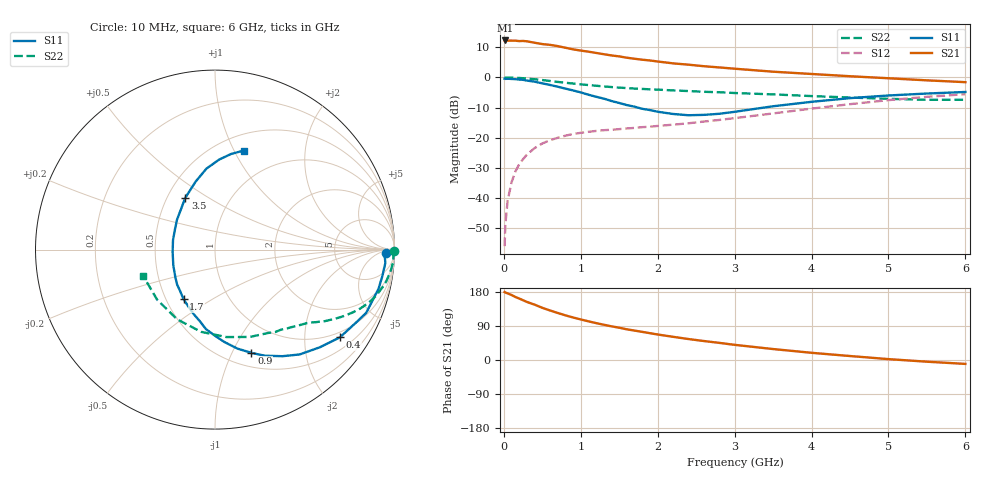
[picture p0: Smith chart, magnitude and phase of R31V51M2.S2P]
! SIEMENS Small Signal Semiconductors
! BFR181
! Si NPN RF Bipolar Junction Transistor in SOT23
! VCE = 1.5 V  IC = 1.2 mA
! Common Emitter S-Parameters:  May  1996
# GHz  S  MA  R  50
!  f  S11  S21  S12  S22
! GHz  MAG  ANG  MAG  ANG  MAG  ANG  MAG  ANG
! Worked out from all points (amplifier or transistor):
!   36 points, 10 MHz to 6 GHz, reference 50 ohm
!   highest |S21| = 12.3 dB at 20 MHz (marker M1)
!   |S21| within 3 dB of that: start of sweep to 912.8 MHz
!   unconditionally stable (mu >= 1): 1.87 GHz to 3.673 GHz
!   at 250 MHz: K = 0.18, MSG = 19.6 dB, |S12| = -27.1 dB
!   at 1.4 GHz: K = 0.84, MSG = 12.3 dB, |S12| = -17.3 dB
!   at 6 GHz: K = 0.88, MSG = 2.0 dB, |S12| = -5.5 dB
!   S11 on the Smith chart (normalised r, x): 10 MHz: 37, -13; 400 MHz: 0.83, -2.95; 900 MHz: 0.65, -1.19; 1.7 GHz: 0.61, -0.38; 3.5 GHz: 0.62, +0.40; 6 GHz: 0.66, +1.09
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0.01  0.9531 -1.0  4.087 179.4  0.0016 95.8  0.9981 -0.5
0.02  0.946 -1.9  4.1 178.1  0.0037 82.6  0.993 -0.9
0.05  0.9519 -4.5  4.079 175.7  0.0092 88.4  0.9952 -2.2
0.1  0.9442 -8.9  4.075 171.6  0.0183 84.3  0.9942 -4.2
0.15  0.9368 -13.6  4.063 166.2  0.0276 80.1  0.9871 -6.5
0.25  0.9132 -22.7  4.025 157.7  0.0443 75.2  0.9706 -10.5
0.3  0.8867 -27.0  3.966 153.2  0.0527 73.1  0.9578 -12.5
0.4  0.8505 -35.1  3.759 146.1  0.0674 68.3  0.9344 -15.9
0.5  0.7982 -43.0  3.571 137.7  0.0804 64.0  0.9055 -19.1
0.6  0.7507 -51.1  3.465 130.7  0.0913 60.0  0.8744 -22.0
0.7  0.7026 -57.7  3.305 124.2  0.0999 56.7  0.8436 -24.5
0.9  0.6097 -70.6  2.92 112.2  0.1156 51.6  0.7927 -28.4
1.1  0.5175 -84.2  2.672 102.1  0.1256 48.1  0.7476 -31.7
1.4  0.4064 -102.2  2.313 88.8  0.1358 45.3  0.6928 -35.7
1.7  0.3273 -122.4  2.04 77.6  0.1458 45.3  0.6537 -38.9
2  0.2702 -144.7  1.837 67.3  0.1572 45.9  0.6283 -42.4
2.2  0.2481 -159.5  1.711 61.2  0.1649 47.1  0.6093 -45.0
2.8  0.2498 153.3  1.465 45.2  0.1976 49.8  0.569 -53.8
3.5  0.3329 119.8  1.245 28.9  0.2533 50.5  0.5239 -68.3
4.5  0.454 96.0  1.047 10.5  0.3607 44.6  0.4646 -99.6
5.5  0.5412 80.3  0.895 -4.5  0.4773 32.1  0.4265 -139.1
6  0.5744 73.8  0.835 -10.3  0.5286 24.4  0.4259 -159.8
